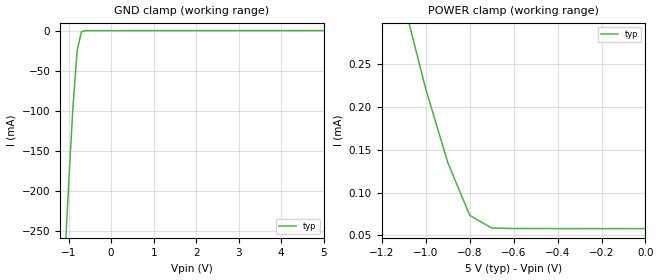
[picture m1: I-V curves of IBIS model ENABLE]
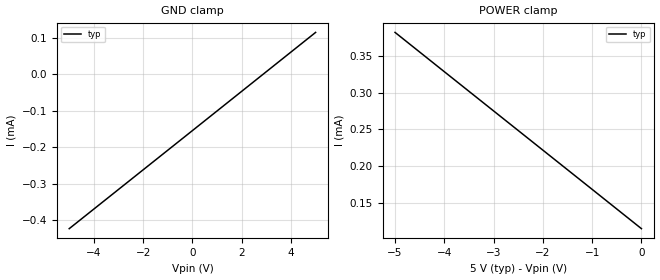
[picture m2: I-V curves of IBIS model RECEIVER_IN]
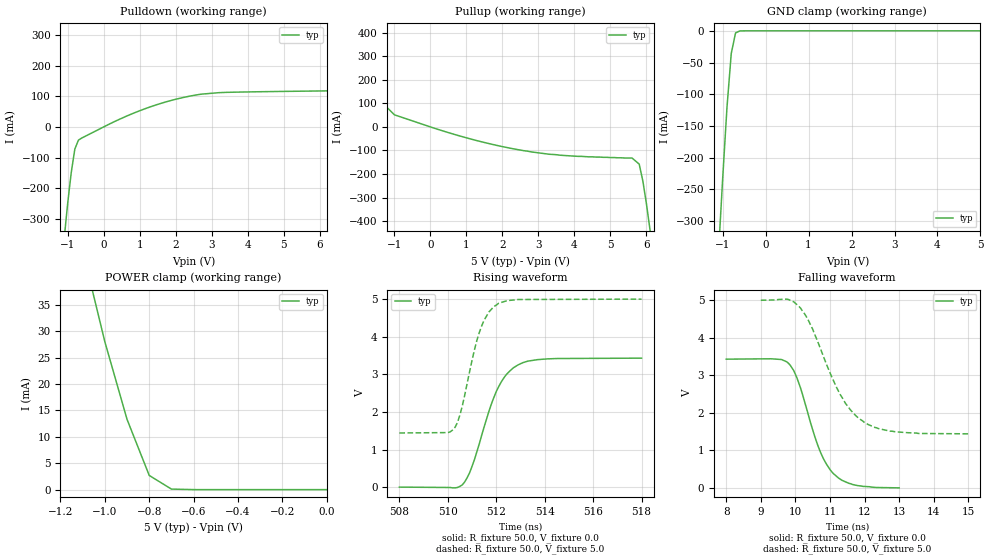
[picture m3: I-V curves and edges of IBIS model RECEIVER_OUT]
|   Texas Instruments Incorporated
|   Data Transmissions Products
|   IBIS Model for SN75LBC175A
|   16D SOIC Package
[IBIS Ver]   3.2
[Comment char]   |_char
[File name]   lbc175ad.ibs
[File Rev]   2.0
[Date]   8Jan01
[Source]   File originated at Texas Instruments Incorporated.
   Data Transmission Products Group. All data based on
   Bench Measurements.
[Notes]
[Disclaimer]
(C) Copyright Texas Instruments Incorporated 2001
   All rights reserved
  Texas Instruments Incorporated hereby grants the user of this IBIS
model a non-exclusive, nontransferable license to use this IBIS model
under the following terms.  Before using this IBIS model, the user
should read this license.  If the user does not accept these terms,
the IBIS model should be returned to Texas Instruments within 30 days.
  The user is granted this license only to use the IBIS model and
is not granted rights to sell, load, rent, lease or license the IBIS
model in whole or in part, or in modified form to anyone other than
user.  User may modify the IBIS model to suit its specific applications
but rights to derivative works and such modifications shall belong to
Texas Instruments.
  This IBIS model is provided on an "AS IS" basis and Texas Instruments
makes absolutely no warranty with respect to the information contained
herein.  TEXAS INSTRUMENTS DISCLAIMS AND CUSTOMER WAIVES ALL WARRANTIES,
EXPRESS OR IMPLIED, INCLUDING WARRANTIES OF MERCHANTABILITY OR FITNESS
FOR A PARTICULAR PURPOSE. The entire risk as to quality and performance
is with the Customer. ACCORDINGLY, IN NO EVENT SHALL THE COMPANY BE LIABLE
FOR ANY DAMAGES, WHETHER IN CONTRACT OR TORT,INCLUDING ANY LOST PROFITS
OR OTHER INCIDENTAL, CONSEQUENTIAL, EXEMPLARY, OR PUNITIVE DAMAGES ARISING
OUT OF THE USE OR APPLICATION OF THE IBIS model provided in this package.
Further, Texas Instruments reserves the right to discontinue or make changes
without notice to any product herein to improve reliability, function, or
design. Texas Instruments does not convey any license under patent rights
or any other intellectual property rights, including those of third parties.
Contact Texas Instruments at ATTN:DATA TRANSMISSIONS
[Copyright]   Copyright 2001, Texas Instruments, All Rights Reserved
[Component]   SN75LBC175AD
[Manufacturer]  Texas Instruments Incorporated
[Package]
|   typ   min   max
R_pkg   0.035   0.030   0.040
L_pkg   2.181nH   1.231nH   3.257nH
C_pkg   0.322pF   0.163pF   0.546pF
[Pin]   signal_name   model_name   R_pin   L_pin   C_pin
1   1B   RECEIVER_IN   0.040   3.251n   0.546p
2   1A   RECEIVER_IN   0.039   2.561n   0.393p
3   1Y   RECEIVER_OUT   0.030   1.681n   0.186p
4   1,2EN   ENABLE   0.030   1.231n   0.163p
5   2Y   RECEIVER_OUT   0.030   1.231n   0.163p
6   2A   RECEIVER_IN   0.030   1.681n   0.186p
7   2B   RECEIVER_IN   0.039   2.564n   0.393p
8   GND   GND   0.040   3.257n   0.545p
9   3B   RECEIVER_IN   0.040   3.247n   0.546p
10   3A   RECEIVER_IN   0.039   2.558n   0.394p
11   3Y   RECEIVER_OUT   0.030   1.681n   0.187p
12   3,4EN   ENABLE   0.030   1.231n   0.163p
13   4Y   RECEIVER_OUT   0.030   1.231n   0.163p
14   4A   RECEIVER_IN   0.030   1.681n   0.187p
15   4B   RECEIVER_IN   0.039   2.558n   0.394p
16   VCC   POWER   0.040   3.246n   0.546p
[Diff_pin]   inv_pin   vdiff   tdelay_typ   tdelay_min   tdelay_max
| The 'xA' pin is Diff_pin and the 'xB' pin is the inv_pin
2   1   200mV   0 0 0   | Vth  +/-200mV
6   7   200mV   0 0 0
10   9   200mV   0 0 0
14   15   200mV   0 0 0
| Models and submodels in the file (3): ENABLE (Input), RECEIVER_IN (Input), RECEIVER_OUT (3-state)
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|   Receiver Enable Model
[Model]   ENABLE
Model_type   Input
|Signals   1,2EN,3,4EN
Vinh = 2.0
Vinl = 0.8
|   typ   min   max
C_comp   1.0pF   NA   NA
|   typ   min   max
[Temperature Range]   25.0   NA   NA
[Voltage range]   5.0V   4.75V   5.25V
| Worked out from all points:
|   GND clamp passes 1 mA (typ) near -0.67 V on its own axis
[GND_clamp]
|   Voltage   I(typ)   I(min)   I(max)
-5V       -4.21A     NA         NA
-2V       -1.22A     NA         NA
-1V       -192mA     NA         NA
-900mV    -96.1mA    NA         NA
-800mV    -24.8mA    NA         NA
-700mV    -1.47mA    NA         NA
-500mV    -17.2uA    NA         NA
5V        57.8uA     NA         NA
[Power_clamp]
| Note that the[POWER_clamp]voltage table is referenced to Vcc
| and is calculated using Vtable=Vcc - Vmeasured.
|   Voltage   I(typ)   I(min)   I(max)
-5V       4.391mA    NA         NA
-2V       1.232mA    NA         NA
-1V       221.2uA    NA         NA
-900mV    135.3uA    NA         NA
-800mV    73.39uA    NA         NA
-700mV    58.53uA    NA         NA
0V        57.8uA     NA         NA
|   Receiver Input Model
[Model]   RECEIVER_IN
Model_type   Input
|Signals   1A,1B,2A,2B,3A,3B,4A,4B
Vinh = 2.0
Vinl = 0.8
|   typ   min   max
C_comp   1.0pF   NA   NA
|   typ   min   max
[Temperature Range]   25.0   NA   NA
[Voltage range]   5.0V   4.75V   5.25V
[GND_clamp]
|   Voltage   I(typ)   I(min)   I(max)
-5V       -422.5uA   NA         NA
0V        -154.3uA   NA         NA
5V        114.3uA    NA         NA
[Power_clamp]
| Note that the[POWER_clamp]voltage table is referenced to Vcc
| and is calculated using Vtable=Vcc - Vmeasured.
|   Voltage   I(typ)   I(min)   I(max)
-5V       382.5uA    NA         NA
-4V       328.8uA    NA         NA
-3V       275.2uA    NA         NA
-2V       221.6uA    NA         NA
-1V       168uA      NA         NA
0V        114.3uA    NA         NA
|   Receiver Output Model
[Model]   RECEIVER_OUT
Model_type   3-state
| Signals   1Y,2Y,3Y,4Y
Vmeas = 1.5V   |Reference voltage for timing measurements
Cref = 15pF   |Timing specification test load capacitance value
Vref = 0   |Timing specification test load voltage; GND
| variable   typ   min   max
C_comp   1.0pF   NA   NA
|   typ   min   max
[Temperature Range]   25.0   NA   NA
[Voltage range]   5.0V   4.75V   5.25V
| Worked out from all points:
|   slope of the pulldown table from 0 to 0.75 V, typ, clamps not added: 18.3 ohm
|   slope of the pullup table from 0 to 0.75 V, typ, clamps not added: 21.1 ohm
|   GND clamp passes 1 mA (typ) near -0.63 V on its own axis
|   POWER clamp passes 1 mA (typ) near -0.73 V on its own axis
|   rising waveform, R_fixture 50.0, V_fixture 0.0: 20-80 % time 1.09ns typ, NA min, NA max; typ from 0 V to 3.43 V
|   falling waveform, R_fixture 50.0, V_fixture 0.0: 20-80 % time 747ps typ, NA min, NA max; typ from 3.43 V to 0 V
|   rising waveform, R_fixture 50.0, V_fixture 5.0: 20-80 % time 802ps typ, NA min, NA max; typ from 1.44 V to 5 V
|   falling waveform, R_fixture 50.0, V_fixture 5.0: 20-80 % time 1.06ns typ, NA min, NA max; typ from 5 V to 1.44 V
[Pulldown]
|   Voltage   I(typ)   I(min)   I(max)
-5V       -4.96A     NA         NA
-2V       -1.44A     NA         NA
-1V       -251mA     NA         NA
-900mV    -149mA     NA         NA
-800mV    -72.1mA    NA         NA
-700mV    -43mA      NA         NA
400mV     22.9mA     NA         NA
2.7V      107mA      NA         NA
6.3V      118mA      NA         NA
6.6V      139mA      NA         NA
7.7V      328mA      NA         NA
10V       741mA      NA         NA
[Pullup]
|   Voltage   I(typ)   I(min)   I(max)
| Note that the[Pullup]voltage table is referenced to Vcc
| and is calculated using Vtable=Vcc - Vmeasured.
-5V       740mA      NA         NA
-4V       560mA      NA         NA
-3V       380mA      NA         NA
-2V       202mA      NA         NA
-1V       51.4mA     NA         NA
2.4V      -95.6mA    NA         NA
5.6V      -132mA     NA         NA
5.8V      -158mA     NA         NA
5.9V      -229mA     NA         NA
6V        -326mA     NA         NA
7V        -1.44A     NA         NA
10V       -4.96A     NA         NA
| Output in High Impedance (off)
[GND_clamp]
|   Voltage   I(typ)   I(min)   I(max)
-5V       -4.96A     NA         NA
-2V       -1.44A     NA         NA
-1V       -233mA     NA         NA
-900mV    -121mA     NA         NA
-800mV    -35.7mA    NA         NA
-700mV    -3.28mA    NA         NA
-600mV    -151uA     NA         NA
5V        66.5pA     NA         NA
[POWER_clamp]
|   Voltage   I(typ)   I(min)   I(max)
| Note that the [POWER_clamp] voltage table is referenced to Vcc
| and is calculated using Vtable = Vcc - Vmeasured.
| Outputs in Tri-state.
-5V       740mA      NA         NA
-2V       201mA      NA         NA
-1V       28mA       NA         NA
-900mV    13.3mA     NA         NA
-800mV    2.68mA     NA         NA
-700mV    98.5uA     NA         NA
0V        66.5pA     NA         NA
[Ramp]
|   typ   min   max
dV/dt_r   2.54v/1.2ns   NA   NA
dV/dt_f   2.14v/1.0ns   NA   NA
R_load = 50Ohm
[Rising Waveform]
R_fixture = 50.0
V_fixture = 0.0
C_fixture = 0p
L_fixture = 0n
|   V(typ)   V(min)   V(max)
508ns     0V         NA         NA
510.3ns   -20mV      NA         NA
510.6ns   60mV       NA         NA
511ns     550mV      NA         NA
511.7ns   2.02V      NA         NA
512ns     2.54V      NA         NA
512.4ns   2.98V      NA         NA
512.9ns   3.25V      NA         NA
514.1ns   3.41V      NA         NA
518ns     3.43V      NA         NA
[Falling Waveform]
R_fixture = 50.0
V_fixture = 0.0
C_fixture = 0p
L_fixture = 0n
|   V(typ)   V(min)   V(max)
8ns       3.43V      NA         NA
9.3ns     3.44V      NA         NA
9.75ns    3.36V      NA         NA
9.95ns    3.13V      NA         NA
10.05ns   2.92V      NA         NA
10.65ns   1.13V      NA         NA
10.85ns   710mV      NA         NA
11.05ns   430mV      NA         NA
11.65ns   90mV       NA         NA
13ns      0V         NA         NA
[Rising Waveform]
R_fixture = 50.0
V_fixture = 5.0
C_fixture = 0p
L_fixture = 0n
|   V(typ)   V(min)   V(max)
508ns     1.44V      NA         NA
510ns     1.45V      NA         NA
510.3ns   1.59V      NA         NA
510.6ns   2.16V      NA         NA
511.1ns   3.65V      NA         NA
511.3ns   4.11V      NA         NA
511.7ns   4.66V      NA         NA
512.1ns   4.89V      NA         NA
512.9ns   4.99V      NA         NA
518ns     5V         NA         NA
[Falling Waveform]
R_fixture = 50.0
V_fixture = 5.0
C_fixture = 0p
L_fixture = 0n
|   V(typ)   V(min)   V(max)
9ns       5V         NA         NA
9.75ns    5.03V      NA         NA
10.15ns   4.79V      NA         NA
10.5ns    4.23V      NA         NA
11.05ns   2.96V      NA         NA
11.3ns    2.48V      NA         NA
11.6ns    2.07V      NA         NA
12ns      1.74V      NA         NA
12.75ns   1.51V      NA         NA
15ns      1.44V      NA         NA
